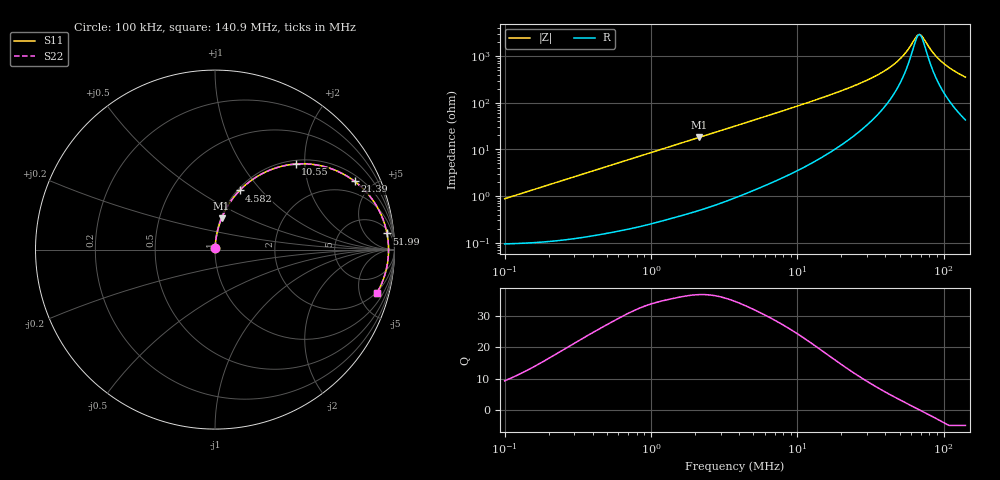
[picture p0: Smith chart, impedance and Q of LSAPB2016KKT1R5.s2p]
! LSAPB2016KKT1R5  S-PARAMETER MODEL  ( General Type )
! Model Generated by TAIYO YUDEN Corporation (http://www.ty-top.com)
! Version 2.0
! TAIYO YUDEN Control No. 20210629
! Copyright(c) 2015 TAIYO YUDEN CO.,LTD. All Rights Reserved.
! Product Description (link to TY-COMPAS)
! https://ds.yuden.co.jp/TYCOMPAS/or/detail?pn=LSAPB2016KKT1R5M&u=M
! Products Name : Inductors
! Characteristics :
!  Inductance : 1.5 uH , SRF(min) : -Hz , DC Resistance(max) : 0.105 Ohm
!  Rated Current : Saturation :2100 mA , Temp Rise : 1800 mA (40 degC)
!  Case Size : 2.0 x 1.6 / 0.079 x 0.063 [mm/inch] , Thickness : 1 / 0.039 [mm/inch]
!  (Conditions: Temperature = 25 degC , DC Bias Current/Voltage = 0A / 0V)
! External Node Assignments :
!  1  o---GGG---o  2
! GND o---------o GND
! Frequency Range : 0.1MHz  -  140.89697MHz  [ 402 STEP ]
# MHz S RI R 50
! Freq[MHz].  S11 Real  S11 Imag  S21 Real  S21 Imag  S12 Real  S12 Imag  S22 Real  S22 Imag
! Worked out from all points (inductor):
!   401 points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, 100 kHz to 140.9 MHz, reference 50 ohm
!   read as one part in series: L = 1.38 uH near 103.7 kHz
!   highest Q = 36.8 at 2.14 MHz (marker M1), where L = 1.35 uH
!   self-resonance near 68.26 MHz
!   S11 on the Smith chart (normalised r, x): 100 kHz: 1.00, +0.02; 4.582 MHz: 1.02, +0.77; 10.55 MHz: 1.08, +1.80; 21.39 MHz: 1.29, +3.91; 51.99 MHz: 7, +18; 140.9 MHz: 1.86, -7.06
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0.1  0.00101 0.00868  0.999 -0.00868  0.999 -0.00868  0.00101 0.00868
0.336853  0.00213 0.029  0.9979 -0.029  0.9979 -0.029  0.00213 0.029
1.134703  0.012 0.0954  0.988 -0.0954  0.988 -0.0954  0.012 0.0954
2.139986  0.0363 0.1738  0.9637 -0.1738  0.9637 -0.1738  0.0363 0.1738
3.753625  0.0978 0.283  0.9022 -0.283  0.9022 -0.283  0.0978 0.283
4.5819  0.1372 0.3293  0.8628 -0.3293  0.8628 -0.3293  0.1372 0.3293
6.827083  0.2564 0.4197  0.7436 -0.4197  0.7436 -0.4197  0.2564 0.4197
10.54798  0.449 0.4767  0.551 -0.4767  0.551 -0.4767  0.449 0.4767
12.64421  0.54 0.4753  0.46 -0.4753  0.46 -0.4753  0.54 0.4753
21.38884  0.7774 0.3808  0.2226 -0.3808  0.2226 -0.3808  0.7774 0.3808
31.29713  0.8889 0.2613  0.1111 -0.2613  0.1111 -0.2613  0.8889 0.2613
42.59248  0.9402 0.1572  0.0598 -0.1572  0.0598 -0.1572  0.9402 0.1572
51.99094  0.9582 0.0903  0.0418 -0.0903  0.0418 -0.0903  0.9582 0.0903
56.92315  0.9631 0.0601  0.0369 -0.0601  0.0369 -0.0601  0.9631 0.0601
64.62413  0.9666 0.0181  0.0334 -0.0181  0.0334 -0.0181  0.9666 0.0181
67.00994  0.9669 0.00611  0.0331 -0.00611  0.0331 -0.00611  0.9669 0.00611
69.48383  0.9669 -0.00587  0.0331 0.00587  0.0331 0.00587  0.9669 -0.00587
72.04905  0.9667 -0.0179  0.0333 0.0179  0.0333 0.0179  0.9667 -0.0179
84.81615  0.9617 -0.072  0.0383 0.072  0.0383 0.072  0.9617 -0.072
94.561  0.9548 -0.1083  0.0452 0.1083  0.0452 0.1083  0.9548 -0.1083
113.3534  0.9365 -0.1695  0.0635 0.1695  0.0635 0.1695  0.9365 -0.1695
140.897  0.9014 -0.2435  0.0986 0.2435  0.0986 0.2435  0.9014 -0.2435
